PROGRAM DININGROOM
VAR	
	fbLight1: FB_Light;
	fbLight2: FB_Light;
	fbLight3: FB_Light;
	
	R_TRIG_BlindUp1: R_TRIG;	
	R_TRIG_BlindDown1: R_TRIG;
	bSwitchBlindUp1: BOOL;
	bSwitchBlindDown1: BOOL;
	fbVenetianBlind1: FB_VenetianBlind;	
	
	R_TRIG_BlindUp2: R_TRIG;	
	R_TRIG_BlindDown2: R_TRIG;
	bSwitchBlindUp2: BOOL;
	bSwitchBlindDown2: BOOL;
	fbVenetianBlind2: FB_VenetianBlind;	
END_VAR
VAR_OUTPUT
	rTemperature: LREAL;
END_VAR

// Light 1
fbLight1(bOn:= , bOff:= , bToggle:= GVL.I_bTerm2_Var1, bLight=> GVL.Q_bTerm3_Var12);

// Light 2
fbLight2(bOn:= , bOff:= , bToggle:= GVL.I_bTerm2_Var2, bLight=> GVL.Q_bTerm3_Var13);
	
// Light 3
fbLight3(bOn:= , bOff:= , bToggle:= GVL.I_bTerm2_Var3, bLight=> GVL.Q_bTerm3_Var14);

	
// Blind 1
R_TRIG_BlindUp1(CLK:=GVL.I_bTerm2_Var4);
bSwitchBlindUp1:=R_TRIG_BlindUp1.Q;
R_TRIG_BlindDown1(CLK:=GVL.I_bTerm2_Var5);
bSwitchBlindDown1:= R_TRIG_BlindDown1.Q;

fbVenetianBlind1(
	bUp:= bSwitchBlindUp1, 
	bDown:= bSwitchBlindDown1, 
	bStop:= (bSwitchBlindUp1 OR bSwitchBlindDown1) AND (fbVenetianBlind1.bBlindUp OR fbVenetianBlind1.bBlindDown), 
	bSwitchOverUp:= , 
	bSwitchOverDown:= , 
	tSwitchOverTime:= , 
	bStepUp:= , 
	bStepDown:= , 
	tStepTime:= , 
	bShadowPosition:= , 
	tShadowTurnAroundTime:= , 
	tShadowTurnOffTime:= , 
	bSafetyPosition:= , 
	tTurnOffTime:= , 
	tSwitchOverDeadTime:= , 
	bBlindUp=> GVL.Q_bTerm9_Var1, 
	bBlindDown=> GVL.Q_bTerm9_Var2);
	
// Blind 2
R_TRIG_BlindUp2(CLK:=GVL.I_bTerm2_Var6);
bSwitchBlindUp2:=R_TRIG_BlindUp2.Q;
R_TRIG_BlindDown2(CLK:=GVL.I_bTerm2_Var7);
bSwitchBlindDown2:= R_TRIG_BlindDown2.Q;

fbVenetianBlind2(
	bUp:= bSwitchBlindUp2, 
	bDown:= bSwitchBlindDown2, 
	bStop:= (bSwitchBlindUp2 OR bSwitchBlindDown2) AND (fbVenetianBlind2.bBlindUp OR fbVenetianBlind2.bBlindDown), 
	bSwitchOverUp:= , 
	bSwitchOverDown:= , 
	tSwitchOverTime:= , 
	bStepUp:= , 
	bStepDown:= , 
	tStepTime:= , 
	bShadowPosition:= , 
	tShadowTurnAroundTime:= , 
	tShadowTurnOffTime:= , 
	bSafetyPosition:= , 
	tTurnOffTime:= , 
	tSwitchOverDeadTime:= , 
	bBlindUp=> GVL.Q_bTerm10_Var1, 
	bBlindDown=> GVL.Q_bTerm10_Var2);
	
// Temperature
rTemperature := INT_TO_LREAL(GVL.I_nTerm5_Var3) / 10;

END_PROGRAM
